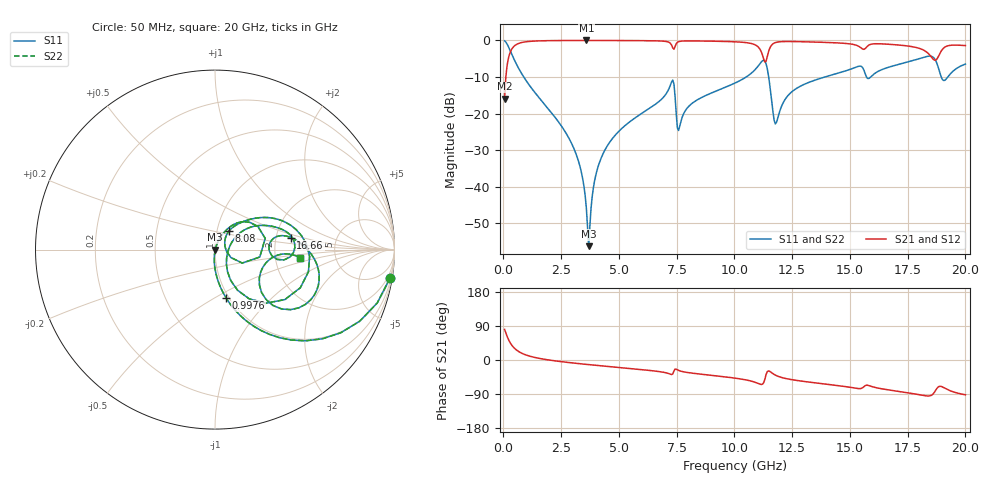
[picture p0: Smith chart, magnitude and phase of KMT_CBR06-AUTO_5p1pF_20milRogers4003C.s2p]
! Data measured by Modelithics Inc. support@modelithics.com 813-866-6335
! KEMET CBR06-AUTO 5.1pF, Pad Width= 0.851mm, Pad Length= 0.64mm, Pad Gap= 0.62mm, 20mil Rogers 4003C substrate Data, January 2022
# hz S ma R 50
! 2 Port Network Data from SP1.SP block
! freq  magS11  angS11  magS21  angS21  magS12  angS12  magS22  angS22
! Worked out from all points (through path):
!   401 points, 50 MHz to 20 GHz, reference 50 ohm
!   highest |S21| = -0.01 dB at 3.591 GHz (marker M1); lowest = -15.9 dB at 50 MHz (marker M2)
!   group delay of S21, straight-line fit = 15.2 ps
!   lowest |S11| = -56.3 dB at 3.691 GHz (marker M3), VSWR 1.00, Z = 50.2 - j0.0293 ohm
!   |S11| at or under -10 dB: 878 MHz to 10.51 GHz (9.632 GHz wide, 169 % of centre); 11.48 GHz to 13.92 GHz (2.435 GHz wide, 19.2 % of centre); 18.95 GHz to 19.24 GHz (286.1 MHz wide, 1.5 % of centre)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
!   |S22| runs from -56.3 to -0.1 dB; largest |S21 - S12| = 0
!   S11 on the Smith chart (normalised r, x): 50 MHz: 1, -12; 997.6 MHz: 0.97, -0.57; 8.08 GHz: 1.14, +0.24; 16.66 GHz: 2.42, +0.40; 20 GHz: 2.77, -0.32
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5e7  0.9872 -9.3  0.1595 80.6  0.1595 80.6  0.9872 -9.3
3.4925e8  0.6598 -49.8  0.7507 40.1  0.7507 40.1  0.6598 -49.8
9.97625e8  0.2771 -77.0  0.9599 12.8  0.9599 12.8  0.2771 -77.0
2.74325e9  0.05178 -94.6  0.9972 -6.1  0.9972 -6.1  0.05178 -94.6
3.391625e9  0.01485 -94.6  0.9983 -10.4  0.9983 -10.4  0.01485 -94.6
3.591125e9  0.005023 -84.0  0.9983 -11.6  0.9983 -11.6  0.005023 -84.0
3.690875e9  0.001539 -10.9  0.9983 -12.2  0.9983 -12.2  0.001539 -10.9
3.990125e9  0.01403 69.5  0.9982 -14.0  0.9982 -14.0  0.01403 69.5
4.439e9  0.03371 70.5  0.9976 -16.6  0.9976 -16.6  0.03371 70.5
6.73325e9  0.1461 57.3  0.9836 -30.5  0.9836 -30.5  0.1461 57.3
7.281875e9  0.2716 28.5  0.8612 -38.4  0.8612 -38.4  0.2716 28.5
7.631e9  0.06724 36.5  0.9695 -28.5  0.9695 -28.5  0.06724 36.5
8.079875e9  0.1308 53.0  0.9842 -34.0  0.9842 -34.0  0.1308 53.0
1.0025e10  0.2613 40.4  0.957 -47.8  0.957 -47.8  0.2613 40.4
1.127188e10  0.5351 -13.3  0.5505 -59.3  0.5505 -59.3  0.5351 -13.3
1.18205e10  0.07554 1.2  0.9426 -41.3  0.9426 -41.3  0.07554 1.2
1.336662e10  0.2776 28.8  0.9515 -59.3  0.9515 -59.3  0.2776 28.8
1.665838e10  0.428 9.0  0.8866 -78.7  0.8866 -78.7  0.428 9.0
1.670825e10  0.4329 8.6  0.8846 -79.2  0.8846 -79.2  0.4329 8.6
1.870325e10  0.5378 -38.5  0.5344 -80.9  0.5344 -80.9  0.5378 -38.5
1.910225e10  0.2844 -19.9  0.8064 -74.2  0.8064 -74.2  0.2844 -19.9
2e10  0.475 -5.5  0.85 -91.9  0.85 -91.9  0.475 -5.5
